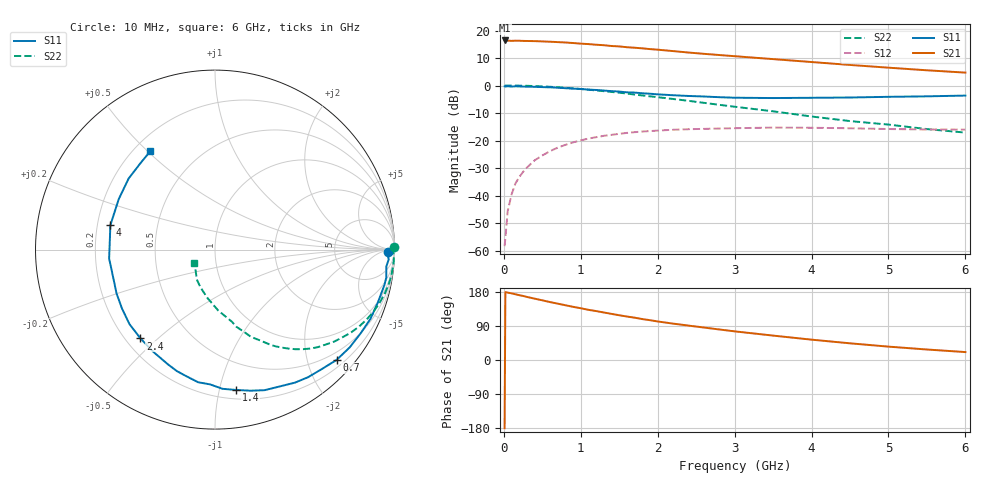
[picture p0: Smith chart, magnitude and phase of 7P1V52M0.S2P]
! Infineon Technologies  Discrete & RF Semiconductors
! BFP620
! SiGe NPN RF Grounded Emitter Transistor in SOT343
! VCE = 1.5 V  IC = 2 mA
! Common Emitter S-Parameters:  February  2000
# GHz  S  MA  R  50
!  f  S11  S21  S12  S22
! GHz  MAG  ANG  MAG  ANG  MAG  ANG  MAG  ANG
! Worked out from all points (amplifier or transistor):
!   36 points, 10 MHz to 6 GHz, reference 50 ohm
!   highest |S21| = 16.4 dB at 10 MHz (marker M1)
!   |S21| within 3 dB of that: start of sweep to 1.848 GHz
!   unconditionally stable (mu >= 1): 5.403 GHz to end of sweep
!   at 250 MHz: K = 0.01, MSG = 23.8 dB, |S12| = -31.4 dB
!   at 1.4 GHz: K = 0.20, MSG = 16.1 dB, |S12| = -17.9 dB
!   at 6 GHz: K = 1.09, MAG = 8.5 dB, |S12| = -16.0 dB
!   lowest NFmin = 0.59 dB at 900 MHz
!   S11 on the Smith chart (normalised r, x): 10 MHz: 50, -20; 700 MHz: 0.34, -2.55; 1.4 GHz: 0.27, -1.13; 2.4 GHz: 0.26, -0.44; 4 GHz: 0.25, +0.11; 6 GHz: 0.26, +0.51
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0.01  0.9664 -0.8  6.599 -180.0  0.0012 84.1  0.9999 0.7
0.02  0.9581 -1.0  6.505 179.3  0.0017 82.1  0.992 -0.8
0.05  0.9695 -3.2  6.54 177.8  0.0052 96.9  0.9975 -1.8
0.1  0.9593 -5.6  6.49 175.9  0.0104 87.7  0.9979 -3.5
0.15  0.9671 -9.2  6.529 173.5  0.0165 85.1  0.9963 -5.4
0.4  0.9481 -24.0  6.42 161.9  0.0436 77.8  0.9777 -14.4
0.6  0.9274 -36.0  6.259 152.9  0.0641 71.0  0.9485 -21.4
0.7  0.9147 -42.2  6.159 148.7  0.0743 67.6  0.93 -24.8
0.9  0.88 -53.9  5.924 140.3  0.0926 60.3  0.8867 -31.5
1.1  0.8428 -64.9  5.67 132.4  0.1086 53.9  0.8402 -37.5
1.3  0.8105 -75.9  5.411 125.4  0.1218 48.0  0.7896 -43.5
1.4  0.7909 -81.4  5.23 121.7  0.127 45.1  0.7642 -46.2
1.5  0.7768 -86.9  5.142 118.1  0.1322 42.8  0.7407 -48.5
1.8  0.7235 -102.7  4.743 108.0  0.1457 35.0  0.6599 -55.8
2.2  0.6658 -120.9  4.229 96.0  0.157 27.2  0.5695 -63.2
2.4  0.6459 -130.0  3.98 90.8  0.1605 23.4  0.5269 -67.5
3  0.6005 -155.9  3.415 75.6  0.1675 14.9  0.4117 -76.9
3.5  0.5919 -175.2  3.022 64.4  0.1719 8.5  0.3399 -87.0
4  0.5986 166.8  2.675 53.7  0.1706 2.8  0.2735 -98.7
4.5  0.6056 152.3  2.368 44.0  0.167 -1.8  0.2257 -111.0
5.5  0.6358 130.8  1.893 27.7  0.1588 -6.4  0.1614 -131.7
6  0.6565 123.2  1.717 20.9  0.1579 -7.4  0.1393 -146.3
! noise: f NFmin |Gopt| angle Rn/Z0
0.9  0.59  0.57  23  0.29
1.8  0.7  0.28  73  0.22
2.4  0.79  0.27  89  0.16
3  1.01  0.29  119  0.13
4  1.16  0.37  167  0.06
5  1.59  0.41  -153  0.1
6  1.79  0.48  -119  0.22
